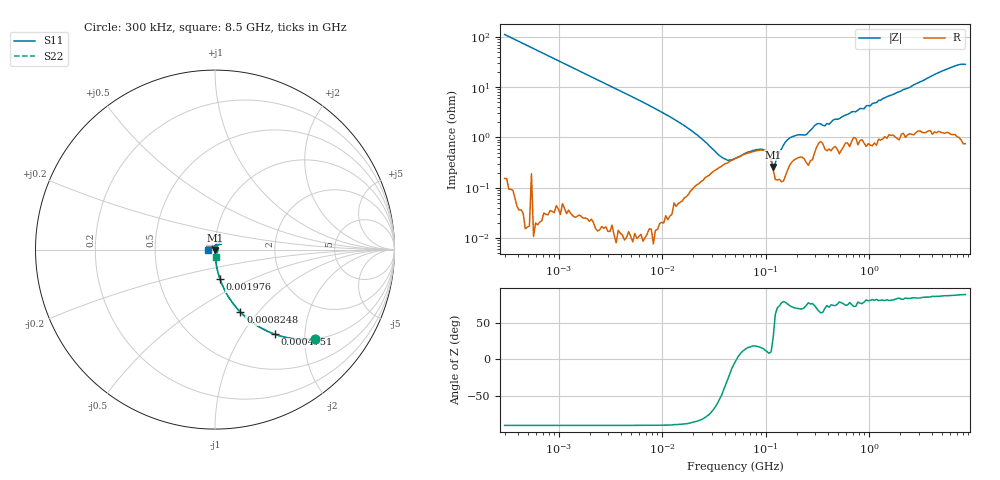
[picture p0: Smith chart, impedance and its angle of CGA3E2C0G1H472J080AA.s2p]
! S-parameter Generated by TDK Corporation
! Copyright(C) 2015 TDK Corporation.
! All Rights Reserved.
! TDK P/N: CGA3E2C0G1H472J080AA (Multilayer Ceramic Chip Capacitors)
! Property: C=4.7nF
! Size(LxWxT): 1.6x0.8x0.8mm, 0.063x0.031x0.031inches
! Model Type: s2p (Touchstone File Format Version 1.0)
! Frequency: DC=Yes Start=0.3MHz Stop=8500MHz 225points Log-sweep
! Note:
! Model Generated on Jun. 23, 2015
! Hash(MD5):
! Port Assignments:
!  1 ---| |--- 2
! Applicable Conditions:
!  Temperature = 25 degC
!  DC Bias Voltage = 0 V
!  Small Signal Operation
! Terms and conditions regarding TDK Simulation Models
! (1)This simulation model is being provided solely for informational purposes. Please refer to the specifications of the products in terms of detailed characteristics of such products.
! (2)In no event shall TDK Corporation of any of its subsidiaries be liable for any loss or damage arising, directly or indirectly,
!  From any information contained in this simulation model, including, but not limited to loss or damages arising from any inaccuracies, omissions or errors in connection with such information.
! (3)Any and all copyrights on this simulation model are owned by TDK Corporation.
!  Duplication or redistribution of this simulation model without prior written permission from TDK Corporation is prohibited.
! (4)This simulation model is subject to any modification or change without any prior notice.
! (5)Neither TDK Corporation nor any of its subsidiaries shall make any warranty, express or implied,
!  Including but not limited to the correctness, implied warranties of merchantability and fitness for a particular purpose with respect to this simulation models.
! (6)The use of this simulation model shall be deemed to have consented to the terms and conditions hereof.
# MHz S MA R 50
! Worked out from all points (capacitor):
!   224 points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, 300 kHz to 8.5 GHz, reference 50 ohm
!   read as one part in series: C = 4.74 nF near 314.1 kHz
!   lowest |Z| = 258 mohm at 118.2 MHz (marker M1)
!   series resonance near 52.22 MHz, so ESL is about 2 nH
!   S11 on the Smith chart (normalised r, x): 300 kHz: 1.00, -2.24; 475.1 kHz: 1.00, -1.41; 824.8 kHz: 1.00, -0.81; 1.976 MHz: 1.00, -0.34; 8.5 GHz: 0.92, -0.00
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0.3  0.7455 -41.7  0.6665 48.1  0.6665 48.3  0.7455 -41.8
0.47509  0.5766 -54.8  0.8164 35.2  0.8167 35.3  0.5763 -54.8
0.8248242  0.3765 -67.8  0.9261 22.1  0.9263 22.2  0.3762 -67.8
1.72111  0.191 -78.9  0.9814 11.0  0.9814 11.0  0.1909 -78.9
1.975628  0.167 -80.3  0.9857 9.6  0.9859 9.6  0.167 -80.3
9.430415  0.03399 -88.1  0.9992 1.9  0.9993 1.9  0.03387 -87.5
51.67171  0.001179 -108.9  0.9951 -0.2  0.9954 -0.1  0.007797 -35.7
89.70948  0.0001694 83.2  0.9918 -0.4  0.9921 -0.4  0.009529 -49.9
118.2037  0.001966 -104.3  0.9945 -0.4  0.9946 -0.4  0.007214 -102.8
148.7505  0.002172 -167.7  0.996 -0.8  0.9962 -0.8  0.001024 102.5
283.1228  0.001225 -164.0  0.9902 -1.6  0.9904 -1.6  0.005783 129.5
428.2171  0.002576 -9.1  0.9891 -2.1  0.989 -2.1  0.006583 114.0
491.5417  0.003842 114.8  0.9866 -2.5  0.9867 -2.4  0.001531 -179.9
538.8791  0.003281 119.7  0.9843 -2.5  0.9848 -2.5  0.01017 130.4
710.042  0.003523 10.7  0.9851 -3.2  0.985 -3.2  0.01279 58.0
853.3868  0.005254 69.9  0.9873 -3.9  0.9864 -3.9  0.009377 28.6
893.5346  0.005426 56.7  0.9875 -4.1  0.9865 -4.0  0.002005 -10.0
979.5854  0.007065 82.4  0.9864 -4.5  0.9876 -4.4  0.007061 53.3
1025.67  0.003769 68.7  0.9856 -4.7  0.9866 -4.7  0.001204 144.8
1073.923  0.006862 67.6  0.9855 -4.9  0.987 -4.9  0.01029 98.7
1551.304  0.01137 45.0  0.9818 -7.1  0.9818 -6.9  0.009741 71.5
8500  0.04026 -177.2  0.9785 -36.6  0.9785 -36.6  0.04034 -84.9
